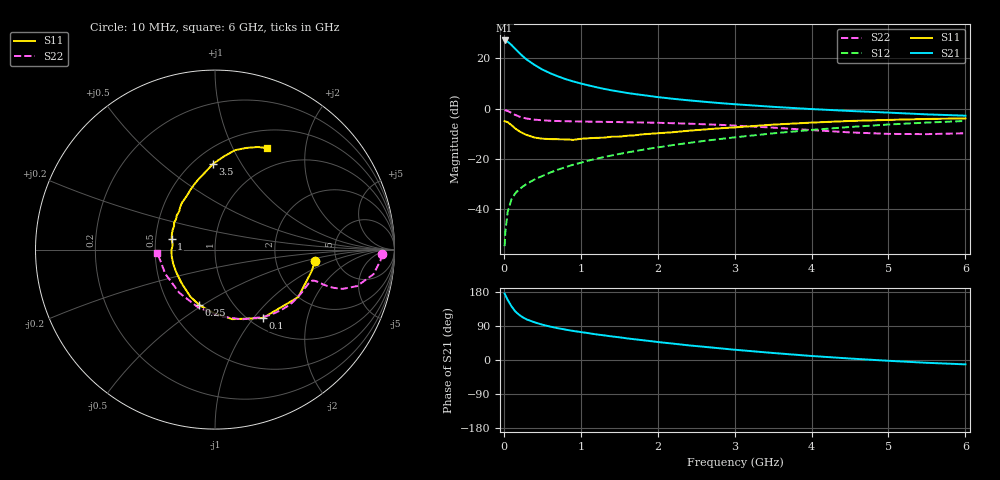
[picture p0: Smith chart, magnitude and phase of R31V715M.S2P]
! SIEMENS Small Signal Semiconductors
! BFR181
! Si NPN RF Bipolar Junction Transistor in SOT23
! VCE = 1.75 V  IC = 15 mA
! Common Emitter S-Parameters:  May  1996
# GHz  S  MA  R  50
!  f  S11  S21  S12  S22
! GHz  MAG  ANG  MAG  ANG  MAG  ANG  MAG  ANG
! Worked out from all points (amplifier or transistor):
!   36 points, 10 MHz to 6 GHz, reference 50 ohm
!   highest |S21| = 27.1 dB at 10 MHz (marker M1)
!   |S21| within 3 dB of that: start of sweep to 137 MHz
!   unconditionally stable (mu >= 1): start of sweep to 11.67 MHz; 336.7 MHz to 3.233 GHz
!   at 250 MHz: K = 0.88, MSG = 25.9 dB, |S12| = -31.1 dB
!   at 1.4 GHz: K = 1.22, MAG = 10.2 dB, |S12| = -18.7 dB
!   at 6 GHz: K = 0.97, MSG = 1.1 dB, |S12| = -5.0 dB
!   S11 on the Smith chart (normalised r, x): 10 MHz: 3.41, -0.63; 100 MHz: 1.15, -1.12; 250 MHz: 0.70, -0.48; 1 GHz: 0.61, +0.08; 3.5 GHz: 0.62, +0.76; 6 GHz: 0.73, +1.38
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0.01  0.5593 -6.5  22.77 175.4  0.0018 89.2  0.9307 -1.6
0.02  0.5532 -12.0  22.49 170.9  0.0035 82.5  0.9246 -3.7
0.05  0.5339 -29.7  21.54 158.7  0.0087 74.7  0.8941 -8.8
0.1  0.4652 -55.0  18.49 141.4  0.0156 70.3  0.8172 -14.4
0.15  0.3993 -76.1  15.35 128.0  0.0205 66.4  0.7443 -17.1
0.2  0.3529 -91.4  12.9 119.1  0.0245 65.9  0.6924 -17.9
0.25  0.3205 -106.0  10.89 112.1  0.028 65.1  0.6558 -18.0
0.3  0.2955 -117.8  9.409 106.8  0.0315 66.2  0.6295 -17.8
0.4  0.2636 -135.1  7.393 99.5  0.0386 67.8  0.5997 -17.4
0.5  0.2505 -149.3  6.001 93.2  0.0451 69.4  0.5821 -17.4
0.6  0.2459 -161.1  5.077 88.3  0.0527 70.7  0.5708 -17.6
0.7  0.2442 -170.4  4.398 84.0  0.0602 71.8  0.5631 -18.2
0.8  0.2425 -179.4  3.873 80.3  0.0677 71.7  0.5581 -18.9
1  0.2488 166.3  3.16 73.7  0.0829 72.7  0.5513 -20.9
1.1  0.2552 160.4  2.895 70.8  0.0916 72.5  0.548 -22.1
1.3  0.2626 150.3  2.468 65.1  0.1077 72.2  0.5416 -24.6
1.6  0.2862 138.1  2.045 57.1  0.1326 71.2  0.533 -28.9
2.2  0.3372 117.9  1.563 43.2  0.1869 67.9  0.5095 -38.9
3.5  0.4773 91.4  1.081 18.5  0.3196 55.5  0.4157 -69.2
4.5  0.565 78.6  0.894 3.9  0.4286 42.4  0.3341 -106.9
5.5  0.6196 67.3  0.764 -7.4  0.5247 27.5  0.3083 -154.1
6  0.6357 62.7  0.72 -11.5  0.5639 19.6  0.3214 -176.7
